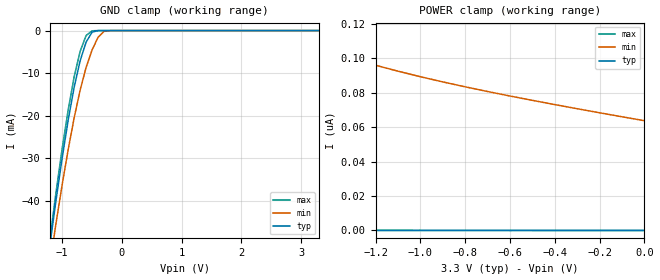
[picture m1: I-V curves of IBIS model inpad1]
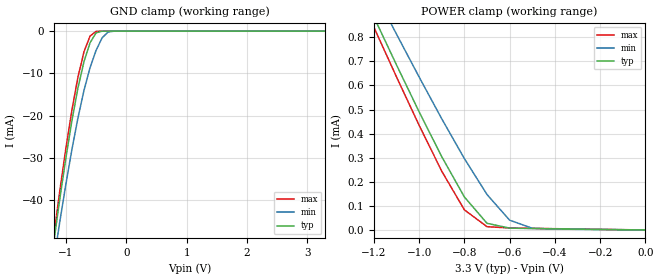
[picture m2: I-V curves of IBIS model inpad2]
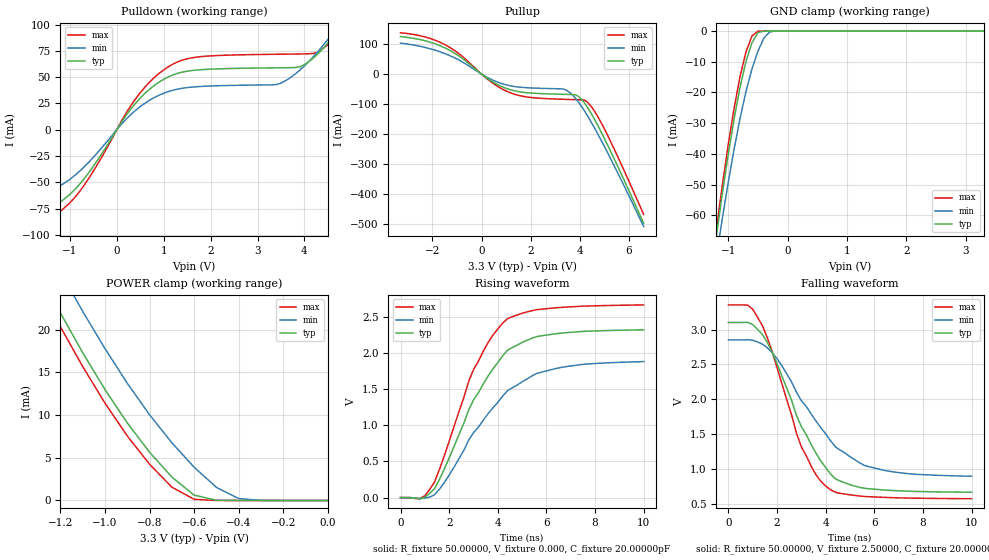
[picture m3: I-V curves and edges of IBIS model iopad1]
| IBIS file 73250bb.ibs created by s2ibis2 version 1.2
| North Carolina State University Electronics Research Laboratory  1995
[IBIS ver]   2.1
[File name]   73250bb.ibs
[File Rev]   1.2
[Date]   11/10/2004
[Source]   Integrated Device Technology, Inc.
[Notes]   1.Temperatures: typ=25C, min=100C, max=0C
   2.Ramp rates based on 50 ohm load.
   3.The model for the open-drain dta pin does not reflect a
   pulsed pull-up device which aides the output on highz.
[Disclaimer] Integrated Device Technology, Inc. ("IDT") hereby grants the
   user of this IBIS model a non-exclusive, nontransferable
   license to use this IBIS model under the following terms. The
   user is granted this license only to use the IBIS model and is
   not granted rights to sell, copy (except as needed to run the
   IBIS model), rent, lease or sub-license the IBIS model in
   whole or in part, or in modified form to anyone. The User may
   modify the IBIS model to suit its specific applications, but
   rights to derivative works and such modifications shall belong
   to IDT. This IBIS model is provided on an AS IS" basis and IDT
   makes absolutely no warranty with respect to the information
   contained herein. IDT DISCLAIMS AND CUSTOMER WAIVES ALL
   WARRANTIES, EXPRESS AND IMPLIED, INCLUDING WARRANTIES OF
   MERCHANTABILITY AND FITNESS FOR A PARTICULAR PURPOSE. THE
   ENTIRE RISK AS TO QUALITY AND PERFORMANCE IS WITH THE USER
   ACCORDINGLY, IN NO EVENT SHALL IDT BE LIABLE FOR ANY DIRECT OR
   INDIRECT DAMAGES, WHETHER IN CONTRACT OR TORT, INCLUDING ANY
   LOST PROFITS OR OTHER INCIDENTAL, CONSEQUENTIAL, EXEMPLARY, OR
   PUNITIVE DAMAGES ARISING OUT OF THE USE OR APPLICATION OF THE
   IBIS model. Further, IDT reserves the right to make changes
   without notice to any product herein to improve reliability,
   function, or design. IDT does not convey any license under
   patent rights or any other intellectual property rights,
   including those of third parties. IDT is not obligated to
   provide maintenance or support for the licensed IBIS model.
[Copyright]   Copyright 2001, Integrated Device Technology, Inc. all rights
   reserved
|   Component 72v73250
[Component]   72v73250
[Manufacturer]   Integrated Device Technology
[Package]
| BB144
| variable   typ   min   max
R_pkg   100.00000m   50.00000m   0.30000
L_pkg   3.00000nH   2.20000nH   4.00000nH
C_pkg   0.70000pF   0.50000pF   0.80000pF
[Pin]   signal_name   model_name   R_pin   L_pin   C_pin
A3   ode   inpad1
A2   resetx   inpad1
A1   clk   inpad1
B1   foi   inpad1
B2   fe_hclk   inpad1
C2   tms   inpad2
C3   tdi   inpad2
D1   tdo   iopad1
D2   tck   inpad1
D3   trstx   inpad2
D4   dsx   inpad1
E1   csx   inpad1
E2   rwx   inpad1
E3   a0   inpad1
F1   a1   inpad1
F2   a2   inpad1
F3   a3   inpad1
G3   a4   inpad1
G2   a5   inpad1
G1   a6   inpad1
H3   a7   inpad1
H2   a8   inpad1
H1   a9   inpad1
J4   a10   inpad1
J3   a11   inpad1
J2   a12   inpad1
J1   a13   inpad1
K3   a14   inpad1
L2   dtax   outpad3
L1   d15   iopad2
M1   d14   iopad2
M2   d13   iopad2
M3   d12   iopad2
L3   d11   iopad2
M4   d10   iopad2
L4   d9   iopad2
K4   d8   iopad2
M5   d7   iopad2
L5   d6   iopad2
K5   d5   iopad2
M6   d4   iopad2
L6   d3   iopad2
K6   d2   iopad2
K7   d1   iopad2
L7   d0   iopad2
G11   rx15   inpad1
G10   rx14   inpad1
F10   rx13   inpad1
F11   rx12   inpad1
F12   rx11   inpad1
E10   rx10   inpad1
E11   rx9   inpad1
E12   rx8   inpad1
A6   rx7   inpad1
C5   rx6   inpad1
B5   rx5   inpad1
A5   rx4   inpad1
C4   rx3   inpad1
B4   rx2   inpad1
A4   rx1   inpad1
B3   rx0   inpad1
K11   tx15   iopad1
J12   tx14   iopad1
J11   tx13   iopad1
J10   tx12   iopad1
H12   tx11   iopad1
H11   tx10   iopad1
H10   tx9   iopad1
G12   tx8   iopad1
A8   tx7   iopad1
B8   tx6   iopad1
C8   tx5   iopad1
A7   tx4   iopad1
B7   tx3   iopad1
C7   tx2   iopad1
C6   tx1   iopad1
B6   tx0   iopad1
E4   vdd   POWER
F4   vdd   POWER
G4   vdd   POWER
H4   vdd   POWER
J5   vdd   POWER
J6   vdd   POWER
J7   vdd   POWER
J8   vdd   POWER
E9   vdd   POWER
F9   vdd   POWER
G9   vdd   POWER
H9   vdd   POWER
D5   vdd   POWER
D6   vdd   POWER
D7   vdd   POWER
D8   vdd   POWER
E5   vss   GND
E6   vss   GND
E7   vss   GND
E8   vss   GND
F5   vss   GND
F6   vss   GND
F7   vss   GND
F8   vss   GND
G5   vss   GND
G6   vss   GND
G7   vss   GND
G8   vss   GND
H5   vss   GND
H6   vss   GND
H7   vss   GND
H8   vss   GND
| in   in   dummy_model
| oe   oe   dummy_model
[Pin Mapping]  pulldown_ref   pullup_ref   gnd_clamp_ref   power_clamp_ref
A3   vss   vdd
A2   vss   vdd
A1   vss   vdd
B1   vss   vdd
B2   vss   vdd
C2   vss   vdd
C3   vss   vdd
D1   vss   vdd
D2   vss   vdd
D3   vss   vdd
D4   vss   vdd
E1   vss   vdd
E2   vss   vdd
E3   vss   vdd
F1   vss   vdd
F2   vss   vdd
F3   vss   vdd
G3   vss   vdd
G2   vss   vdd
G1   vss   vdd
H3   vss   vdd
H2   vss   vdd
H1   vss   vdd
J4   vss   vdd
J3   vss   vdd
J2   vss   vdd
J1   vss   vdd
K3   vss   vdd
L2   vss   vdd
L1   vss   vdd
M1   vss   vdd
M2   vss   vdd
M3   vss   vdd
L3   vss   vdd
M4   vss   vdd
L4   vss   vdd
K4   vss   vdd
M5   vss   vdd
L5   vss   vdd
K5   vss   vdd
M6   vss   vdd
L6   vss   vdd
K6   vss   vdd
K7   vss   vdd
L7   vss   vdd
G11   vss   vdd
G10   vss   vdd
F10   vss   vdd
F11   vss   vdd
F12   vss   vdd
E10   vss   vdd
E11   vss   vdd
E12   vss   vdd
A6   vss   vdd
C5   vss   vdd
B5   vss   vdd
A5   vss   vdd
C4   vss   vdd
B4   vss   vdd
A4   vss   vdd
B3   vss   vdd
K11   vss   vdd
J12   vss   vdd
J11   vss   vdd
J10   vss   vdd
H12   vss   vdd
H11   vss   vdd
H10   vss   vdd
G12   vss   vdd
A8   vss   vdd
B8   vss   vdd
C8   vss   vdd
A7   vss   vdd
B7   vss   vdd
C7   vss   vdd
C6   vss   vdd
B6   vss   vdd
E4   nc   vdd
F4   nc   vdd
G4   nc   vdd
H4   nc   vdd
J5   nc   vdd
J6   nc   vdd
J7   nc   vdd
J8   nc   vdd
E9   nc   vdd
F9   nc   vdd
G9   nc   vdd
H9   nc   vdd
D5   nc   vdd
D6   nc   vdd
D7   nc   vdd
D8   nc   vdd
E5   vss   nc
E6   vss   nc
E7   vss   nc
E8   vss   nc
F5   vss   nc
F6   vss   nc
F7   vss   nc
F8   vss   nc
G5   vss   nc
G6   vss   nc
G7   vss   nc
G8   vss   nc
H5   vss   nc
H6   vss   nc
H7   vss   nc
H8   vss   nc
| Models and submodels in the file (5): inpad1 (Input), inpad2 (Input), iopad1 (3-state), iopad2 (3-state), outpad3 (Open_drain)
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|   Model inpad1
[Model]   inpad1
Model_type   Input
Polarity   Non-Inverting
Vinl =  0.80000V
Vinh =  2.00000V
C_comp   5.00000pF   NA   NA
[Temperature Range]   25.00000   100.00000   0.000
[Voltage Range]   3.30000V   3.00000V   3.60000V
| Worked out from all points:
|   GND clamp passes 1 mA (typ) near -0.53 V on its own axis
[GND_clamp]
| voltage   I(typ)   I(min)   I(max)
-3.3V     -310mA     -295.4mA   -315.4mA
-1.2V     -49.78mA   -54.27mA   -48.33mA
-1.1V     -39.5mA    -44.95mA   -37.65mA
-900mV    -21.04mA   -27.95mA   -18.63mA
-800mV    -13.32mA   -20.5mA    -10.85mA
-700mV    -7.09mA    -13.99mA   -4.876mA
-600mV    -2.698mA   -8.653mA   -1.161mA
-500mV    -374.6uA   -4.55mA    -53.22uA
-400mV    -11.83uA   -1.585mA   -1.231uA
-300mV    -285.2nA   -196.8uA   -25.38nA
-200mV    -6.527nA   -10.13uA   -459.3pA
3.3V      26.9pA     70.7nA     2.066pA
[POWER_clamp]
| voltage   I(typ)   I(min)   I(max)
-3.3V     3.879nA    456nA      684.6pA
-3V       2.36nA     327.1nA    413.6pA
-2.7V     1.415nA    242.1nA    246pA
-1.7V     242.2pA    118.8nA    39.53pA
-1.6V     203.7pA    113.3nA    32.78pA
-1.5V     171.8pA    108.3nA    27.21pA
-1.3V     123.7pA    99.68nA    18.83pA
-1.2V     105.8pA    95.94nA    15.74pA
-1V       78.71pA    89.29nA    11.07pA
-800mV    60.2pA     83.42nA    7.956pA
-600mV    47.4pA     78.08nA    5.874pA
0V        26.91pA    63.75nA    2.762pA
|   Model inpad2
[Model]   inpad2
Model_type   Input
Polarity   Non-Inverting
Vinl =  0.80000V
Vinh =  2.00000V
C_comp   5.00000pF   NA   NA
[Temperature Range]   26.00000   100.00000   0.000
[Voltage Range]   3.30000V   3.00000V   3.60000V
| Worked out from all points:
|   GND clamp passes 1 mA (typ) near -0.52 V on its own axis
|   POWER clamp passes 1 mA (typ) near -1.26 V on its own axis
[GND_clamp]
| voltage   I(typ)   I(min)   I(max)
-3.3V     -309.8mA   -295.4mA   -315.4mA
-1.2V     -49.84mA   -54.27mA   -48.33mA
-1.1V     -39.57mA   -44.95mA   -37.66mA
-900mV    -21.14mA   -27.95mA   -18.63mA
-800mV    -13.42mA   -20.5mA    -10.85mA
-700mV    -7.183mA   -13.99mA   -4.88mA
-600mV    -2.772mA   -8.654mA   -1.172mA
-500mV    -409.4uA   -4.553mA   -66.79uA
-400mV    -23.35uA   -1.589mA   -14.97uA
-300mV    -10.73uA   -203.7uA   -13.76uA
-200mV    -10.42uA   -17.24uA   -13.74uA
3.3V      29.82pA    2.653uA    -3.476uA
[POWER_clamp]
| voltage   I(typ)   I(min)   I(max)
-3.3V     5.268mA    4.958mA    5.394mA
-1.2V     884.9uA    994.3uA    842.3uA
-1.1V     685.6uA    813.3uA    635.7uA
-1V       490.6uA    635.3uA    434.7uA
-900mV    304.4uA    461.6uA    244uA
-800mV    137uA      296.4uA    83.56uA
-700mV    27.6uA     147.2uA    13.6uA
-600mV    7.666uA    40.58uA    8.253uA
-500mV    5.845uA    7.214uA    6.75uA
0V        29.82pA    63.75nA    2.762pA
|   Model iopad1
[Model]   iopad1
Model_type   3-state
Polarity   Non-Inverting
Enable   Active-High
|Vinl =  0.80000V
|Vinh =  2.00000V
Vmeas =  1.50000V
C_comp   5.00000pF   NA   NA
[Temperature Range]   25.00000   100.00000   0.000
[Voltage Range]   3.30000V   3.00000V   3.60000V
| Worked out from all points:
|   slope of the pulldown table from 0 to 0.495 V, typ, clamps not added: 16.6 ohm
|   slope of the pullup table from 0 to 0.495 V, typ, clamps not added: 17.8 ohm
|   GND clamp passes 1 mA (typ) near -0.51 V on its own axis
|   POWER clamp passes 1 mA (typ) near -0.62 V on its own axis
|   rising waveform, R_fixture 50.00000, V_fixture 0.000, C_fixture 20.00000pF: 20-80 % time 2.08ns typ, 2.41ns min, 1.83ns max; typ from 0 V to 2.32 V
|   falling waveform, R_fixture 50.00000, V_fixture 2.50000, C_fixture 20.00000pF: 20-80 % time 1.86ns typ, 2.29ns min, 1.6ns max; typ from 3.1 V to 0.664 V
[Pulldown]
| voltage   I(typ)   I(min)   I(max)
-3.3V     -98.4mA    -81.6mA    -110.5mA
-1.9V     -86.7mA    -69mA      -97.4mA
-1.3V     -72.39mA   -56.23mA   -81.63mA
-700mV    -46.93mA   -35.66mA   -53.13mA
500mV     30.12mA    21.95mA    35.15mA
1.3V      53.65mA    38.65mA    64.55mA
3.5V      58.91mA    44.27mA    71.8mA
4V        61.97mA    60.76mA    72.13mA
4.3V      72.71mA    74.98mA    74.18mA
4.7V      93.7mA     97.87mA    90.09mA
4.9V      106.9mA    111.1mA    101.7mA
6.6V      332.3mA    305.7mA    332.7mA
[Pullup]
| voltage   I(typ)   I(min)   I(max)
-3.3V     125.2mA    103.6mA    137.8mA
-2.3V     111.4mA    89.05mA    124mA
-1.5V     87.93mA    68.71mA    98.74mA
400mV     -23.23mA   -17.72mA   -26.94mA
1.2V      -52.73mA   -39.41mA   -63mA
3.3V      -67.33mA   -49.39mA   -83.89mA
3.6V      -67.91mA   -61.92mA   -84.61mA
4V        -78.45mA   -99.51mA   -85.44mA
4.2V      -97.4mA    -124.1mA   -87.42mA
4.5V      -136.2mA   -165.3mA   -111.4mA
5.3V      -265.2mA   -289.4mA   -232.6mA
6.6V      -497.9mA   -508.6mA   -468.4mA
[GND_clamp]
| voltage   I(typ)   I(min)   I(max)
-3.3V     -424.5mA   -403.9mA   -432.6mA
-1.2V     -66.92mA   -73.75mA   -64.72mA
-1.1V     -53.15mA   -61.24mA   -50.45mA
-900mV    -28.53mA   -38.43mA   -25.1mA
-800mV    -18.24mA   -28.42mA   -14.76mA
-700mV    -9.879mA   -19.65mA   -6.761mA
-600mV    -3.823mA   -12.36mA   -1.619mA
-500mV    -522.3uA   -6.579mA   -69.89uA
-400mV    -15.84uA   -2.286mA   -1.491uA
-300mV    -368.6nA   -278.7uA   -29.25nA
-200mV    -8.239nA   -14.25uA   -516.1pA
3.3V      29.26pA    12.72uA    2.135pA
[POWER_clamp]
| voltage   I(typ)   I(min)   I(max)
-3.3V     169.2mA    163.5mA    171.9mA
-1.3V     26.89mA    31.6mA     25.32mA
-1.2V     21.93mA    26.74mA    20.31mA
-1.1V     17.28mA    22.12mA    15.66mA
-1V       12.97mA    17.76mA    11.38mA
-900mV    9.066mA    13.71mA    7.542mA
-800mV    5.637mA    10.02mA    4.237mA
-700mV    2.735mA    6.75mA     1.558mA
-600mV    627uA      3.884mA    134.9uA
-500mV    26.21uA    1.53mA     2.445uA
-400mV    585.2nA    230uA      43.52nA
0V        29.28pA    88.51nA    2.883pA
[Ramp]
| variable   typ   min   max
dV/dt_r   1.39320/1.55145n   1.13040/1.90274n   1.59900/1.32996n
dV/dt_f   1.40130/1.59333n   1.10340/2.00863n   1.61178/1.36973n
R_load = 50.00000
[Rising Waveform]
R_fixture = 50.00000
V_fixture = 0.000
C_fixture = 20.00000pF
R_dut = 100.00000m
L_dut = 3.00000nH
C_dut = 0.70000pF
| time   V(typ)   V(min)   V(max)
0s        0V         0V         0V
800ps     -15.33mV   -14.76mV   -14.41mV
1.4ns     123.7mV    40.45mV    217mV
2ns       545.2mV    310.4mV    777mV
3ns       1.348V     895.9mV    1.767V
3.8ns     1.776V     1.239V     2.242V
4.4ns     2.034V     1.476V     2.47V
5.6ns     2.223V     1.714V     2.595V
6.4ns     2.263V     1.782V     2.62V
10ns      2.316V     1.877V     2.66V
[Falling Waveform]
R_fixture = 50.00000
V_fixture = 2.50000
C_fixture = 20.00000pF
R_dut = 100.00000m
L_dut = 3.00000nH
C_dut = 0.70000pF
| time   V(typ)   V(min)   V(max)
0s        3.103V     2.852V     3.355V
800ps     3.105V     2.855V     3.352V
1.4ns     2.929V     2.791V     3.056V
2ns       2.51V      2.582V     2.454V
3ns       1.606V     1.981V     1.316V
3.6ns     1.225V     1.687V     915.6mV
4ns       1.019V     1.503V     753mV
4.4ns     855.4mV    1.315V     662.5mV
5.6ns     719.8mV    1.048V     602.8mV
10ns      663.6mV    894.1mV    571mV
